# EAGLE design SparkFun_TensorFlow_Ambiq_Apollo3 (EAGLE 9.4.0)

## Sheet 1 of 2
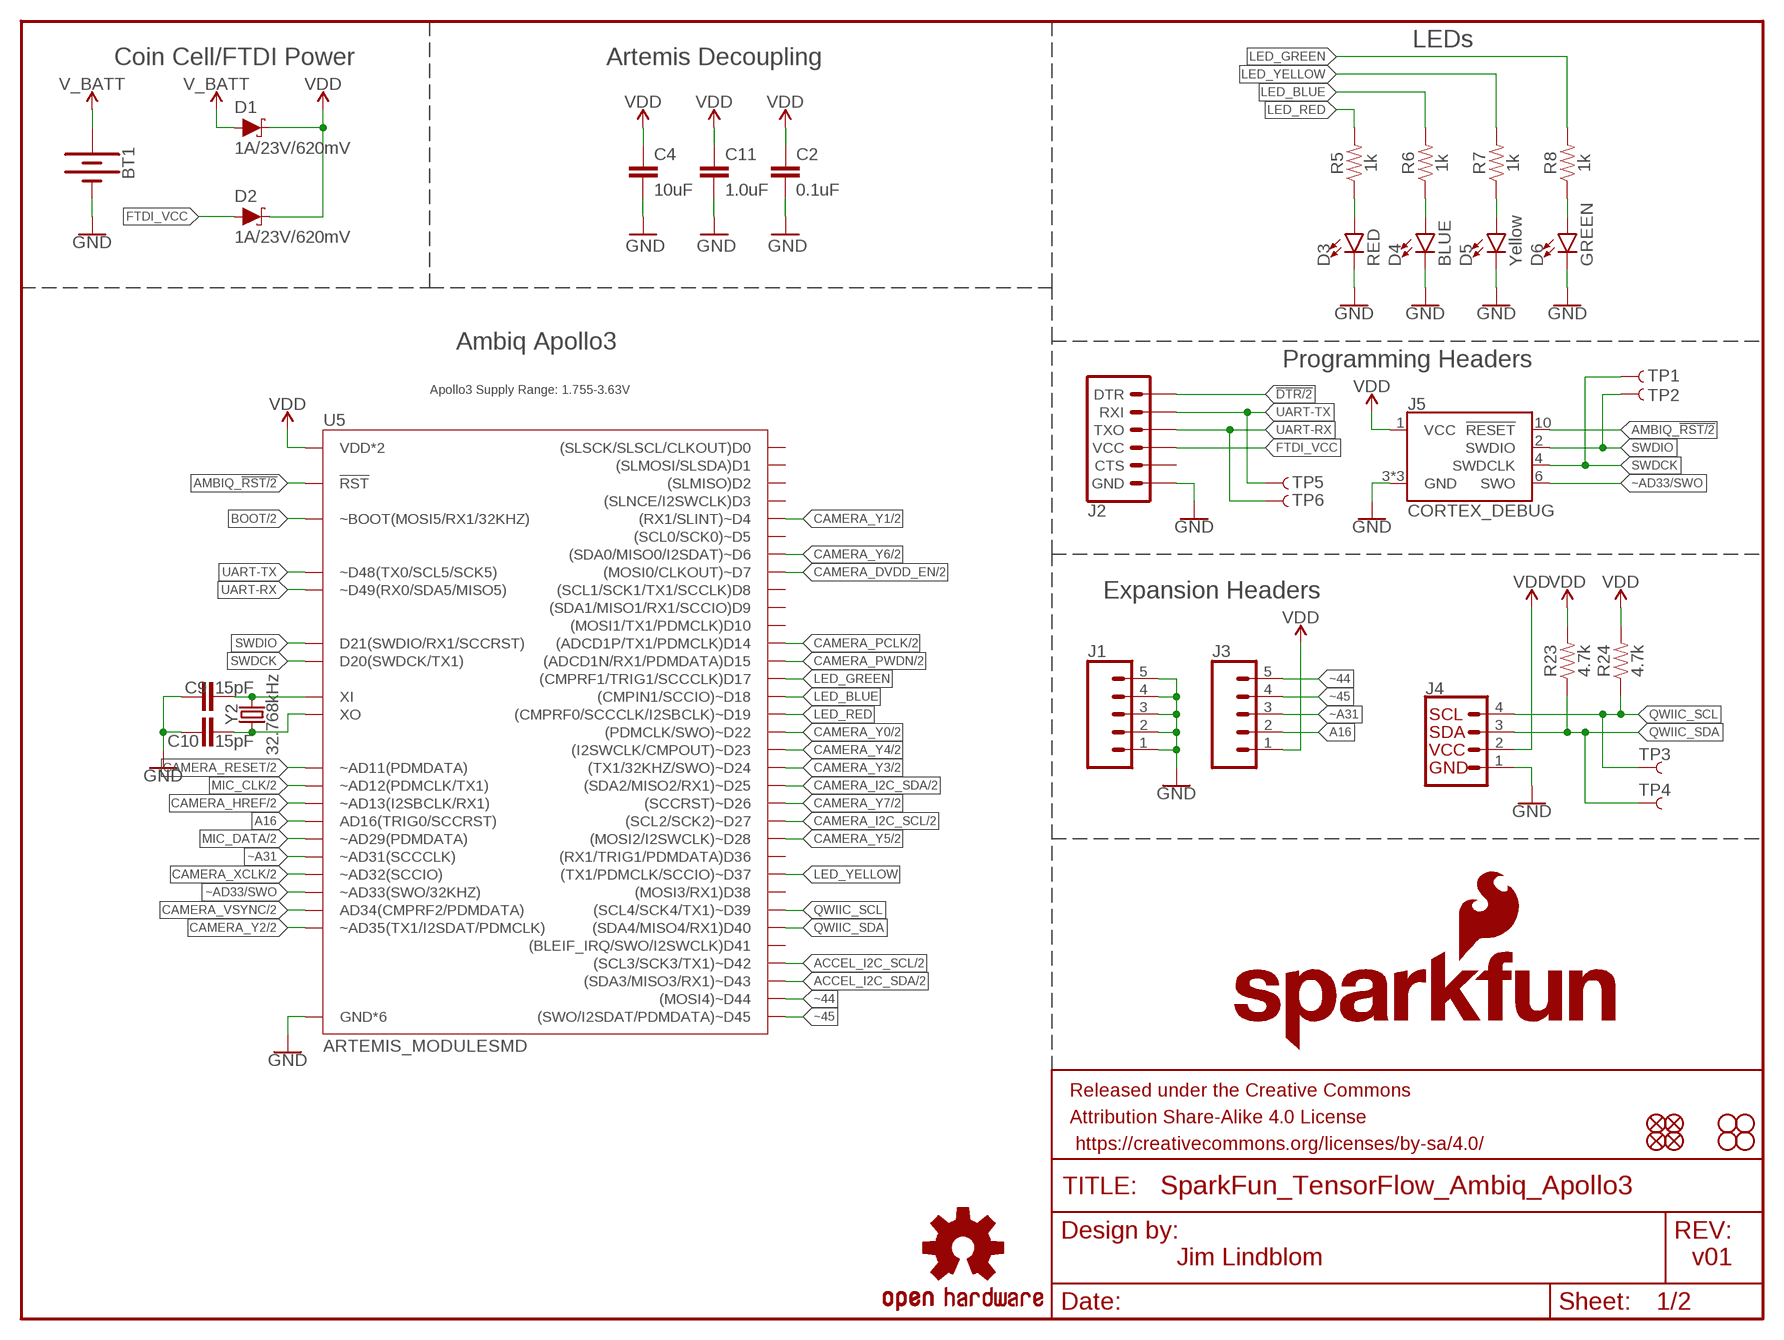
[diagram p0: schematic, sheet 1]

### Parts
BT1  BATTERY-20MM_SMD_4LEGS_OVERPASTE_INNER  [BATTCON_20MM_4LEGS_OVERPASTE_INNER]
C2  0.1uF  0.1UF-0402T-16V-10%  [0402-TIGHT]
C4  10uF  10UF-0603-6.3V-20%  [0603]
C9  15pF  15PF-0402-TIGHT-50V-5%  [0402-TIGHT]
C10  15pF  15PF-0402-TIGHT-50V-5%  [0402-TIGHT]
C11  1.0uF  1.0UF-0402T-16V-10%  [0402-TIGHT]
D1  1A/23V/620mV  DIODE-SCHOTTKY-BAT20J  [SOD-323]
D2  1A/23V/620mV  DIODE-SCHOTTKY-BAT20J  [SOD-323]
D3  RED  LED-RED0603  [LED-0603]
D4  BLUE  LED-BLUE0603  [LED-0603]
D5  Yellow  LED-YELLOW0603  [LED-0603]
D6  GREEN  LED-GREEN0603  [LED-0603]
FD1  FIDUCIAL1X2  [FIDUCIAL-1X2]
FD2  FIDUCIAL1X2  [FIDUCIAL-1X2]
FD3  FIDUCIAL1X2  [FIDUCIAL-1X2]
FD4  FIDUCIAL1X2  [FIDUCIAL-1X2]
FRAME1  FRAME-LETTER  [CREATIVE_COMMONS]
H1  STAND-OFF  [STAND-OFF]
H2  STAND-OFF  [STAND-OFF]
H3  STAND-OFF  [STAND-OFF]
H4  STAND-OFF  [STAND-OFF]
J1  CONN_05NO_SILK  [1X05_NO_SILK]
J2  6_PIN_SERIAL_TARGETSMD  [1X06-SMD_RA_MALE]
J3  CONN_05NO_SILK  [1X05_NO_SILK]
J4  QWIIC_CONNECTORJS-1MM  [JST04_1MM_RA]
J5  CORTEX_DEBUG  CORTEX_DEBUG_MINIMUM_PTH_NS  [2X5-PTH-1.27MM-NO_SILK]
LOGO1  SFE_LOGO_NAME_FLAME.1_INCH  [SFE_LOGO_NAME_FLAME_.1]
LOGO2  OSHW-LOGOS  [OSHW-LOGO-S]
R5  1k  1KOHM-0603-1/10W-1%  [0603]
R6  1k  1KOHM-0603-1/10W-1%  [0603]
R7  1k  1KOHM-0603-1/10W-1%  [0603]
R8  1k  1KOHM-0603-1/10W-1%  [0603]
R23  4.7k  4.7KOHM-0603-1/10W-1%  [0603]
R24  4.7k  4.7KOHM-0603-1/10W-1%  [0603]
TP1  TEST-POINT3X5  [PAD.03X.05]
TP2  TEST-POINT3X5  [PAD.03X.05]
TP3  TEST-POINT3X5  [PAD.03X.05]
TP4  TEST-POINT3X5  [PAD.03X.05]
TP5  TEST-POINT3X5  [PAD.03X.05]
TP6  TEST-POINT3X5  [PAD.03X.05]
U5  ARTEMIS_MODULESMD  [ARTEMIS_FP]
Y2  32.768kHz  CRYSTAL-32.768KHZSMD-3.2X1.5  [CRYSTAL-SMD-3.2X1.5MM]

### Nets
!DTR: J2.1(DTR) ; also sheet 2
A16: J3.2 U5.AD16(AD16(TRIG0/SCCRST))
ACCEL_I2C_SCL: U5.~D42((SCL3/SCK3/TX1)~D42) ; also sheet 2
ACCEL_I2C_SDA: U5.~D43((SDA3/MISO3/RX1)~D43) ; also sheet 2
AMBIQ_!RST: J5.10(!RESET) U5.~RST(!RST) ; also sheet 2
BOOT: U5.BOOT(~BOOT(MOSI5/RX1/32KHZ)) ; also sheet 2
CAMERA_DVDD_EN: U5.D7((MOSI0/CLKOUT)~D7) ; also sheet 2
CAMERA_HREF: U5.~AD13(~AD13(I2SBCLK/RX1)) ; also sheet 2
CAMERA_I2C_SCL: U5.~D27((SCL2/SCK2)~D27) ; also sheet 2
CAMERA_I2C_SDA: U5.~D25((SDA2/MISO2/RX1)~D25) ; also sheet 2
CAMERA_PCLK: U5.D14((ADCD1P/TX1/PDMCLK)D14) ; also sheet 2
CAMERA_PWDN: U5.D15((ADCD1N/RX1/PDMDATA)D15) ; also sheet 2
CAMERA_RESET: U5.~AD11(~AD11(PDMDATA)) ; also sheet 2
CAMERA_VSYNC: U5.AD34(AD34(CMPRF2/PDMDATA)) ; also sheet 2
CAMERA_XCLK: U5.~AD32(~AD32(SCCIO)) ; also sheet 2
CAMERA_Y0: U5.~D22((PDMCLK/SWO)~D22) ; also sheet 2
CAMERA_Y1: U5.~D4((RX1/SLINT)~D4) ; also sheet 2
CAMERA_Y2: U5.~AD35(~AD35(TX1/I2SDAT/PDMCLK)) ; also sheet 2
CAMERA_Y3: U5.~D24((TX1/32KHZ/SWO)~D24) ; also sheet 2
CAMERA_Y4: U5.~D23((I2SWCLK/CMPOUT)~D23) ; also sheet 2
CAMERA_Y5: U5.~D28((MOSI2/I2SWCLK)~D28) ; also sheet 2
CAMERA_Y6: U5.~D6((SDA0/MISO0/I2SDAT)~D6) ; also sheet 2
CAMERA_Y7: U5.~D26((SCCRST)~D26) ; also sheet 2
FTDI_VCC: D2.A J2.4(VCC)
GND: BT1.2(-) C2.1 C4.2 C9.1 C10.1 C11.2 D3.C D4.C D5.C D6.C J1.1 J1.2 J1.3 J1.4 J1.5 J2.6(GND) J4.1 J5.3(GND) J5.5(GND) J5.9(GND) U5.GND@1(GND*6) U5.GND@22(GND*6) U5.GND@38(GND*6) U5.GND@39(GND*6) U5.GND@47(GND*6) U5.GND@59(GND*6) ; also sheet 2
LED_BLUE: R6.2 U5.~D18((CMPIN1/SCCIO)~D18)
LED_GREEN: R8.2 U5.D17((CMPRF1/TRIG1/SCCCLK)D17)
LED_RED: R5.2 U5.~D19((CMPRF0/SCCCLK/I2SBCLK)~D19)
LED_YELLOW: R7.2 U5.~D37((TX1/PDMCLK/SCCIO)~D37)
MIC_CLK: U5.~AD12(~AD12(PDMCLK/TX1)) ; also sheet 2
MIC_DATA: U5.~AD29(~AD29(PDMDATA)) ; also sheet 2
N$2: C9.2 U5.XI Y2.P$2
N$5: D4.A R6.1
N$6: D3.A R5.1
N$7: D5.A R7.1
N$8: D6.A R8.1
QWIIC_SCL: J4.4 R24.1 TP3.P$1 U5.~D39((SCL4/SCK4/TX1)~D39)
QWIIC_SDA: J4.3 R23.1 TP4.P$1 U5.D40((SDA4/MISO4/RX1)D40)
SWDCK: J5.4(SWDCLK) TP1.P$1 U5.SWDCK(D20(SWDCK/TX1))
SWDIO: J5.2(SWDIO) TP2.P$1 U5.SWDIO(D21(SWDIO/RX1/SCCRST))
UART-RX: J2.3(TXO) TP6.P$1 U5.RXI-0(~D49(RX0/SDA5/MISO5))
UART-TX: J2.2(RXI) TP5.P$1 U5.TXO-0(~D48(TX0/SCL5/SCK5))
V_BATT: BT1.1(+) D1.A
VDD: C2.2 C4.1 C11.1 D1.C D2.C J3.1 J4.2 J5.1(VCC) R23.2 R24.2 U5.VDD@36(VDD*2) U5.VDD@37(VDD*2) ; also sheet 2
X0: C10.2 U5.XO Y2.P$1
~44: J3.5 U5.~D44((MOSI4)~D44)
~45: J3.4 U5.~D45((SWO/I2SDAT/PDMDATA)~D45)
~A31: J3.3 U5.~AD31(~AD31(SCCCLK))
~AD33/SWO: J5.6(SWO) U5.~AD33/SWO(~AD33(SWO/32KHZ))
Unconnected: J2.5(CTS) U5.D0((SLSCK/SLSCL/CLKOUT)D0) U5.D1((SLMOSI/SLSDA)D1) U5.D2((SLMISO)D2) U5.D3((SLNCE/I2SWCLK)D3) U5.D8((SCL1/SCK1/TX1/SCCLK)D8) U5.D9((SDA1/MISO1/RX1/SCCIO)D9) U5.D10((MOSI1/TX1/PDMCLK)D10) U5.D36((RX1/TRIG1/PDMDATA)D36) U5.D38((MOSI3/RX1)D38) U5.D41((BLEIF_IRQ/SWO/I2SWCLK)D41) U5.~D5((SCL0/SCK0)~D5)

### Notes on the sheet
- LEDs
- Coin Cell/FTDI Power | Artemis Decoupling
- Ambiq Apollo3
- Programming Headers
- Apollo3 Supply Range: 1.755-3.63V
- Expansion Headers
- Jim Lindblom | v01

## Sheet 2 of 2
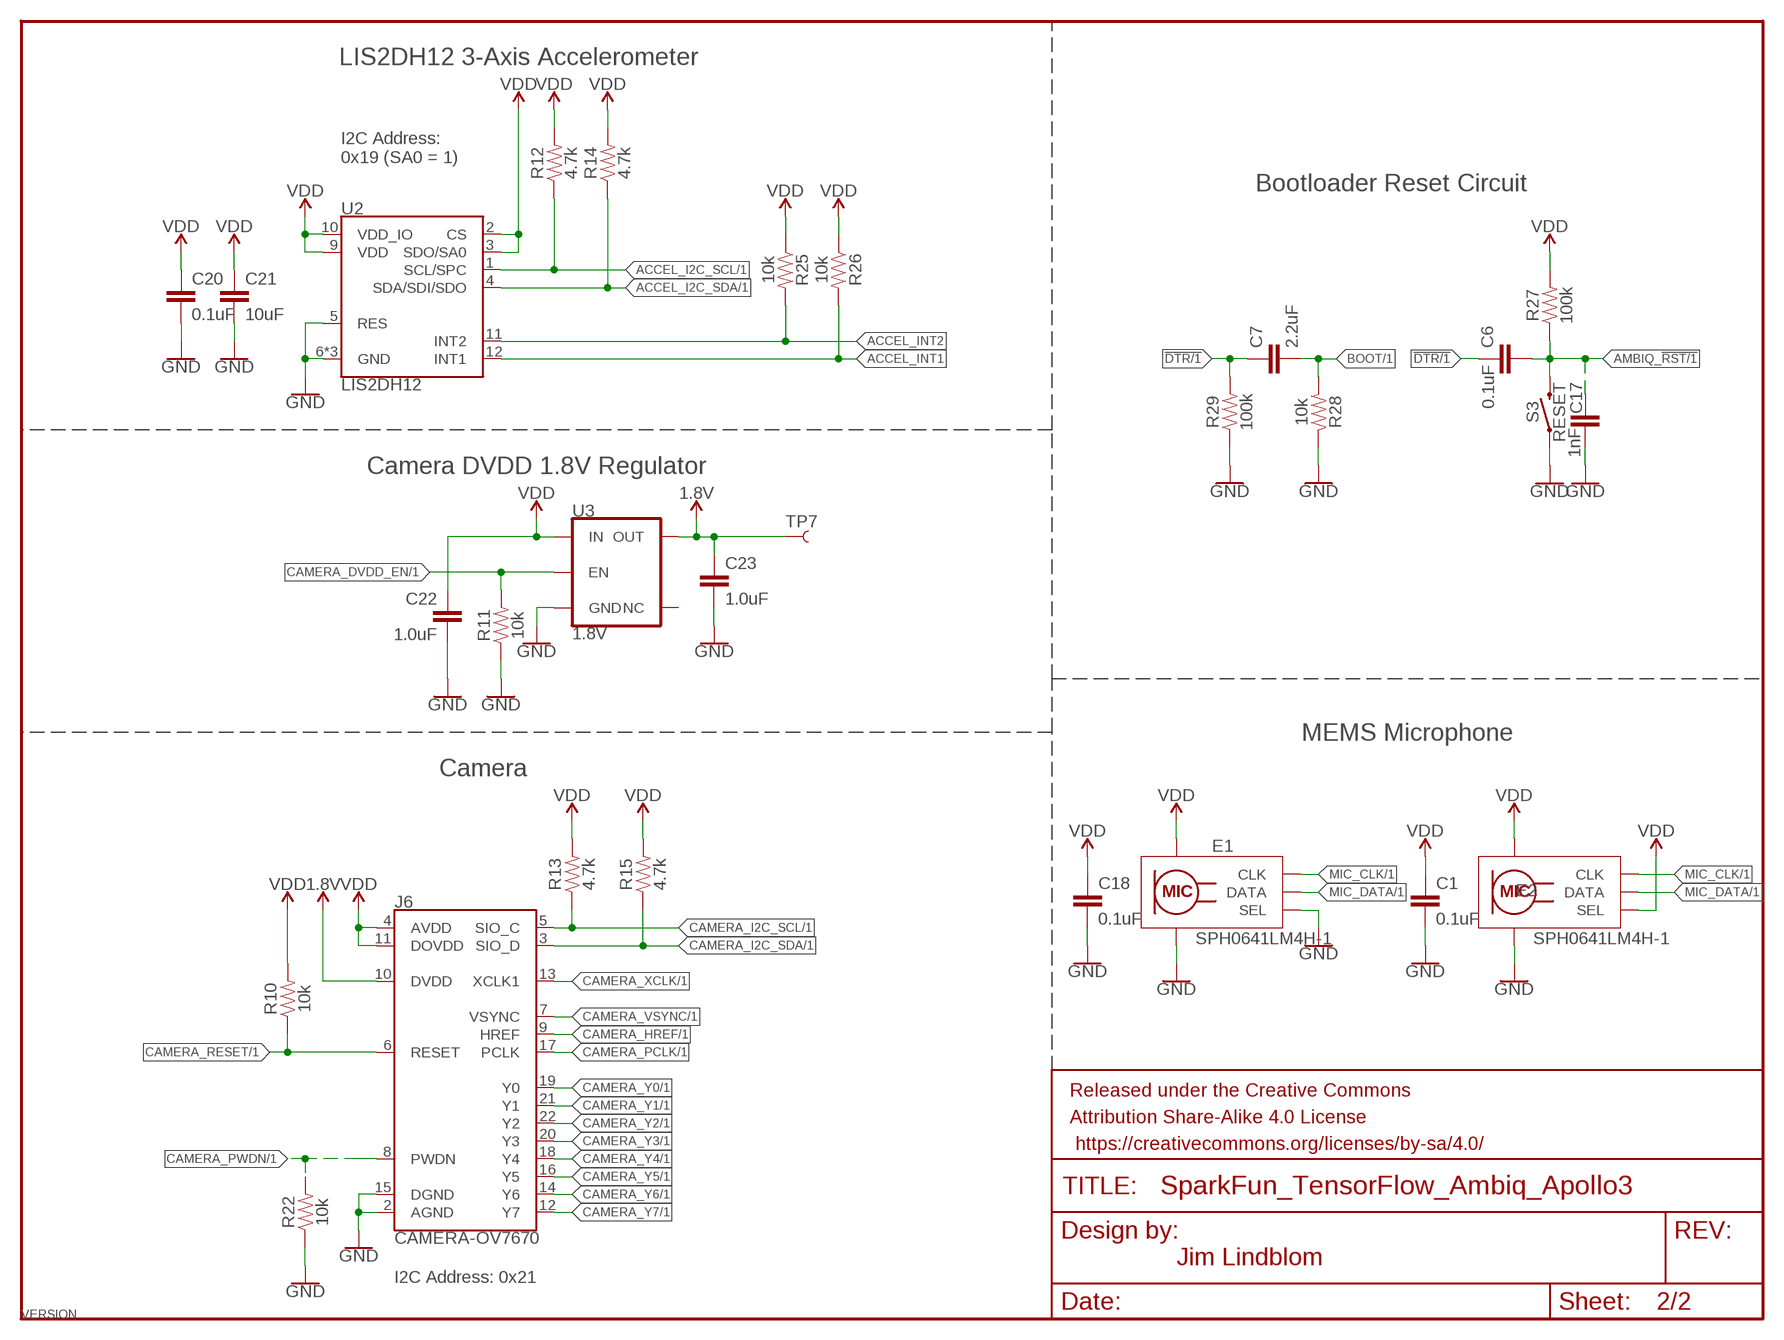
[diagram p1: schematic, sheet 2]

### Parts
C1  0.1uF  0.1UF-0402-TIGHT-16V-10%  [0402-TIGHT]
C6  0.1uF  0.1UF-0603-25V-5%  [0603]
C7  2.2uF  2.2UF-0603-10V-20%  [0603]
C17  1nF  1.0NF/1000PF-0603-50V-10%  [0603]
C18  0.1uF  0.1UF-0402-TIGHT-16V-10%  [0402-TIGHT]
C20  0.1uF  0.1UF-0402-TIGHT-16V-10%  [0402-TIGHT]
C21  10uF  10UF-0603-6.3V-20%  [0603]
C22  1.0uF  1.0UF-0402-TIGHT-16V-10%  [0402-TIGHT]
C23  1.0uF  1.0UF-0402-TIGHT-16V-10%  [0402-TIGHT]
E1  SPH0641LM4H-1  SPH0641LM4H-1_MICROPHONE  [SPH0641LM4H-1_MICROPHONE]
E2  SPH0641LM4H-1  SPH0641LM4H-1_MICROPHONE  [SPH0641LM4H-1_MICROPHONE]
FRAME2  FRAME-LETTERNO_PACKAGE  [DUMMY]
J6  CAMERA-OV7670  [FPC-24-AMPHENOL-SFV24R-1STE1HLF]
R10  10k  10KOHM-0402T-1/16W-1%  [0402-TIGHT]
R11  10k  10KOHM-0402T-1/16W-1%  [0402-TIGHT]
R12  4.7k  4.7KOHM-0603-1/10W-1%  [0603]
R13  4.7k  4.7KOHM-0603-1/10W-1%  [0603]
R14  4.7k  4.7KOHM-0603-1/10W-1%  [0603]
R15  4.7k  4.7KOHM-0603-1/10W-1%  [0603]
R22  10k  10KOHM-0402T-1/16W-1%  [0402-TIGHT]
R25  10k  10KOHM-0402T-1/16W-1%  [0402-TIGHT]
R26  10k  10KOHM-0402T-1/16W-1%  [0402-TIGHT]
R27  100k  100KOHM-0603-1/10W-1%  [0603]
R28  10k  10KOHM-0603-1/10W-1%  [0603]
R29  100k  100KOHM-0603-1/10W-1%  [0603]
S3  RESET  MOMENTARY-SWITCH-SPST-SMD-5.2MM-TALL  [TACTILE_SWITCH_SMD_5.2MM]
TP7  TEST-POINT3X5  [PAD.03X.05]
U2  LIS2DH12  [LGA-12-LISDH12]
U3  1.8V  V_REG_AP2127K-1.8V  [SOT23-5]

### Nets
1.8V: C23.1 J6.10(DVDD) TP7.P$1 U3.5(OUT)
!DTR: C6.1 C7.1 R29.2 ; also sheet 1
ACCEL_I2C_SCL: R12.1 U2.1(SCL/SPC) ; also sheet 1
ACCEL_I2C_SDA: R14.1 U2.4(SDA/SDI/SDO) ; also sheet 1
ACCEL_INT1: R26.2 U2.12(INT1)
ACCEL_INT2: R25.2 U2.11(INT2)
AMBIQ_!RST: C6.2 C17.1 R27.1 S3.3 ; also sheet 1
BOOT: C7.2 R28.2 ; also sheet 1
CAMERA_DVDD_EN: R11.2 U3.3(EN) ; also sheet 1
CAMERA_HREF: J6.9(HREF) ; also sheet 1
CAMERA_I2C_SCL: J6.5(SIO_C) R13.1 ; also sheet 1
CAMERA_I2C_SDA: J6.3(SIO_D) R15.1 ; also sheet 1
CAMERA_PCLK: J6.17(PCLK) ; also sheet 1
CAMERA_PWDN: J6.8(PWDN) R22.2 ; also sheet 1
CAMERA_RESET: J6.6(RESET) R10.1 ; also sheet 1
CAMERA_VSYNC: J6.7(VSYNC) ; also sheet 1
CAMERA_XCLK: J6.13(XCLK1) ; also sheet 1
CAMERA_Y0: J6.19(Y0) ; also sheet 1
CAMERA_Y1: J6.21(Y1) ; also sheet 1
CAMERA_Y2: J6.22(Y2) ; also sheet 1
CAMERA_Y3: J6.20(Y3) ; also sheet 1
CAMERA_Y4: J6.18(Y4) ; also sheet 1
CAMERA_Y5: J6.16(Y5) ; also sheet 1
CAMERA_Y6: J6.14(Y6) ; also sheet 1
CAMERA_Y7: J6.12(Y7) ; also sheet 1
GND: C1.2 C17.2 C18.2 C20.2 C21.2 C22.2 C23.2 E1.2(SEL) E1.3(GND) E1.6(GND) E1.7(GND) E1.8(GND) E2.3(GND) E2.6(GND) E2.7(GND) E2.8(GND) J6.2(AGND) J6.15(DGND) R11.1 R22.1 R28.1 R29.1 S3.1 U2.5(RES) U2.6(GND) U2.7(GND) U2.8(GND) U3.2(GND) ; also sheet 1
MIC_CLK: E1.4(CLK) E2.4(CLK) ; also sheet 1
MIC_DATA: E1.1(DATA) E2.1(DATA) ; also sheet 1
VDD: C1.1 C18.1 C20.1 C21.1 C22.1 E1.5(VDD) E2.2(SEL) E2.5(VDD) J6.4(AVDD) J6.11(DOVDD) R10.2 R12.2 R13.2 R14.2 R15.2 R25.1 R26.1 R27.2 U2.2(CS) U2.3(SDO/SA0) U2.9(VDD) U2.10(VDD_IO) U3.1(IN) ; also sheet 1
Unconnected: J6.MNT1@0(MNT1) J6.MNT1@1(MNT1) J6.MNT2@0(MNT2) J6.MNT2@1(MNT2) U3.4(NC)

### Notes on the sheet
- LIS2DH12 3-Axis Accelerometer
- I2C Address:
  0x19 (SA0 = 1)
- Bootloader Reset Circuit
- Camera DVDD 1.8V Regulator
- MEMS Microphone
- Camera
- Jim Lindblom
- I2C Address: 0x21

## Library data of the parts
BT1 = SparkFun-Batteries:BATTERY: Battery - Single Cell
C1 C18 C20 = ambiq:0.1UF: 0.1µF ceramic capacitors; PROD_ID: CAP-12416
C2 = SparkFun-Capacitors:0.1UF: 0.1µF ceramic capacitors; PROD_ID: CAP-12416
C4 C21 = SparkFun-Capacitors:10UF: 10.0µF ceramic capacitors; PROD_ID: CAP-11015
C6 = SparkFun-Capacitors:0.1UF: 0.1µF ceramic capacitors; PROD_ID: CAP-08604
C7 = SparkFun-Capacitors:2.2UF: 2.2µF ceramic capacitors; PROD_ID: CAP-07888
C9 C10 = ambiq:15PF: 15pF ceramic capacitors; PROD_ID: CAP-13063
C11 = SparkFun-Capacitors:1.0UF: 1µF ceramic capacitors; PROD_ID: CAP-12417
C17 = SparkFun-Capacitors:1.0NF/1000PF: 1nF/1,000pF ceramic capacitors; PROD_ID: CAP-07886
C22 C23 = ambiq:1.0UF: 1µF ceramic capacitors; PROD_ID: CAP-12417
D1 D2 = SparkFun-DiscreteSemi:DIODE-SCHOTTKY: Schottky diode; PROD_ID: DIO-11623
D3 = SparkFun-LED:LED-RED: Red SMD LED; PROD_ID: DIO-00819
D4 = SparkFun-LED:LED-BLUE: Blue SMD LED; PROD_ID: DIO-08575
D5 = SparkFun-LED:LED-YELLOW: Yellow SMD LED; PROD_ID: DIO-09003
D6 = SparkFun-LED:LED-GREEN: Green SMD LED; PROD_ID: DIO-00821
E1 E2 = SparkFun-Sensors:SPH0641LM4H-1_MICROPHONE: SPH0641LM4H-1 Microphone A miniature, high-performance, low power, bottom port silicon digital microphone with a single bit PDM output.; PROD_ID: IC-14361
FD1-FD4 = SparkFun-Aesthetics:FIDUCIAL: Fiducial Alignment Points
FRAME1 = SparkFun-Aesthetics:FRAME-LETTER: Schematic Frame - Letter
FRAME2 = SparkFun-Aesthetics:FRAME-LETTER: Schematic Frame - Letter; DESIGNER: Nobody; VERSION: x01
H1-H4 = SparkFun-Hardware:STAND-OFF: Stand Off
J1 J3 = SparkFun-Connectors:CONN_05: Multi connection point. Often used as Generic Header-pin footprint for 0.1 inch spaced/style header connections On any of the 0.1 inch spaced packages, you can populate with these: Break Away Headers - Straight (PRT-00116) Break Away Male Headers - Right Angle (PRT-00553) Female Headers (PRT-00115)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
J2 = SparkFun-Connectors:6_PIN_SERIAL_TARGET: 6-pin header connection for use with the "FTDI BASIC" pinout - TARGET SIDE. Also known as "Arduino Serial Program Header". It is used to mate with our FTDI Basic serial programmers using the Arduino IDE. Note, this device has "TARGET" in the name. It is intended to be used on a design that contains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; PROD_ID: CONN-08971
J4 = SparkFun-Connectors:QWIIC_CONNECTOR: SparkFun I2C Standard Qwiic Connector An SMD 1mm pitch JST connector makes it easy and quick (get it? Qwiic?) to connect I2C devices to each other. The Qwiic system enables fast and solderless connection between popular platforms and various sensors and actuators. We carry 200mm, 100mm, 50mm, and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; PROD_ID: CONN-13694
J5 = SparkFun-Connectors:CORTEX_DEBUG_MINIMUM: Cortex Debug Connector - 10 pin Supports JTAG debug, Serial Wire debug, and Serial Wire Viewer. PTH and SMD connector options available. General Connector Information Products: PTH Connector -via Digi-Key SparkFun PSoc SparkFun T
J6 = SparkFun-Connectors:CAMERA-OV7670; DIGIKEY: 609-4320-2-ND; PROD_ID: CONN-14233
LOGO1 = SparkFun-Aesthetics:SFE_LOGO_NAME_FLAME: SparkFun Font Logo w/ Flame
LOGO2 = SparkFun-Aesthetics:OSHW-LOGO: Open-Source Hardware (OSHW) Logo
R5-R8 = SparkFun-Resistors:1KOHM: 1kΩ resistor; PROD_ID: RES-07856
R10 R11 R22 R25 R26 = SparkFun-Resistors:10KOHM: 10kΩ resistor; PROD_ID: RES-14241
R12-R15 R23 R24 = SparkFun-Resistors:4.7KOHM: 4.7kΩ resistor; PROD_ID: RES-07857
R27 R29 = SparkFun-Resistors:100KOHM: 100kΩ resistor; PROD_ID: RES-07828
R28 = SparkFun-Resistors:10KOHM: 10kΩ resistor; PROD_ID: RES-00824
S3 = SparkFun-Switches:MOMENTARY-SWITCH-SPST: Momentary Switch (Pushbutton) - SPST; PROD_ID: SWCH-14139
TP1-TP7 = SparkFun-Connectors:TEST-POINT: SparkFun Test Points
U2 = SparkFun-Sensors:LIS2DH12; DIGIKEY: 497-14851-2-ND; PROD_ID: IC-14229
U3 = SparkFun-IC-Power:V_REG_AP2127: AP2127 - 300mA CMOS LDO Regulator w/ Enable The AP2127 is CMOS process low dropout linear regulator with enable function, the regulator delivers a guaranteed 300mA (min.) continuous load current. Features Output Voltage Accuracy: ±1.5% Output Current: 300mA (Min.) Foldback Short Current Protection: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; PROD_ID: VREG-14239
U5 = Testing:ARTEMIS_MODULE
Y2 = SparkFun-Clocks:CRYSTAL-32.768KHZ: 32.768kHz Crystal; PROD_ID: XTAL-13062

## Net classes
0 default: width 0 mm, drill 0 mm
2 usb: width 0.254 mm, drill 0.305 mm, clearance 0.254 mm

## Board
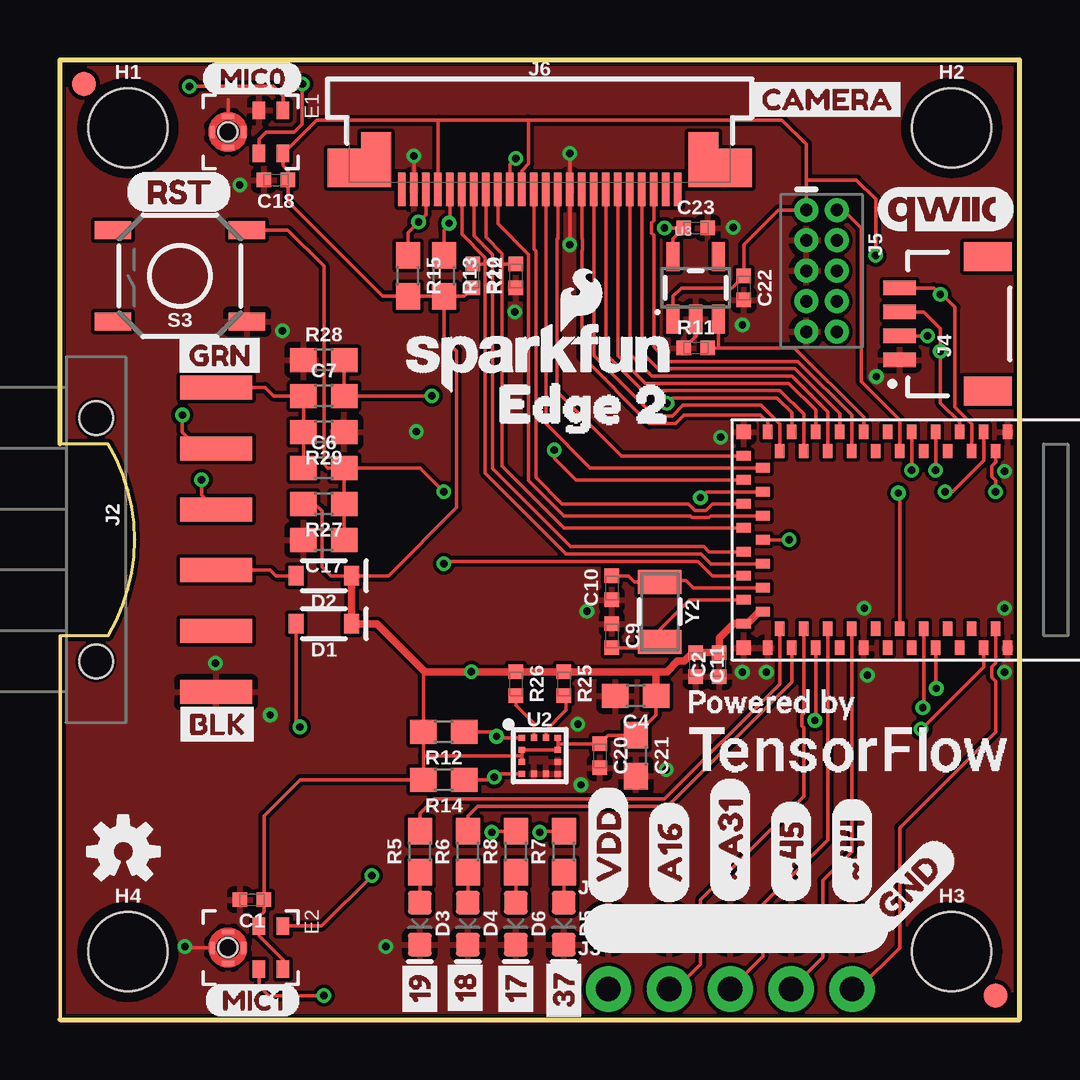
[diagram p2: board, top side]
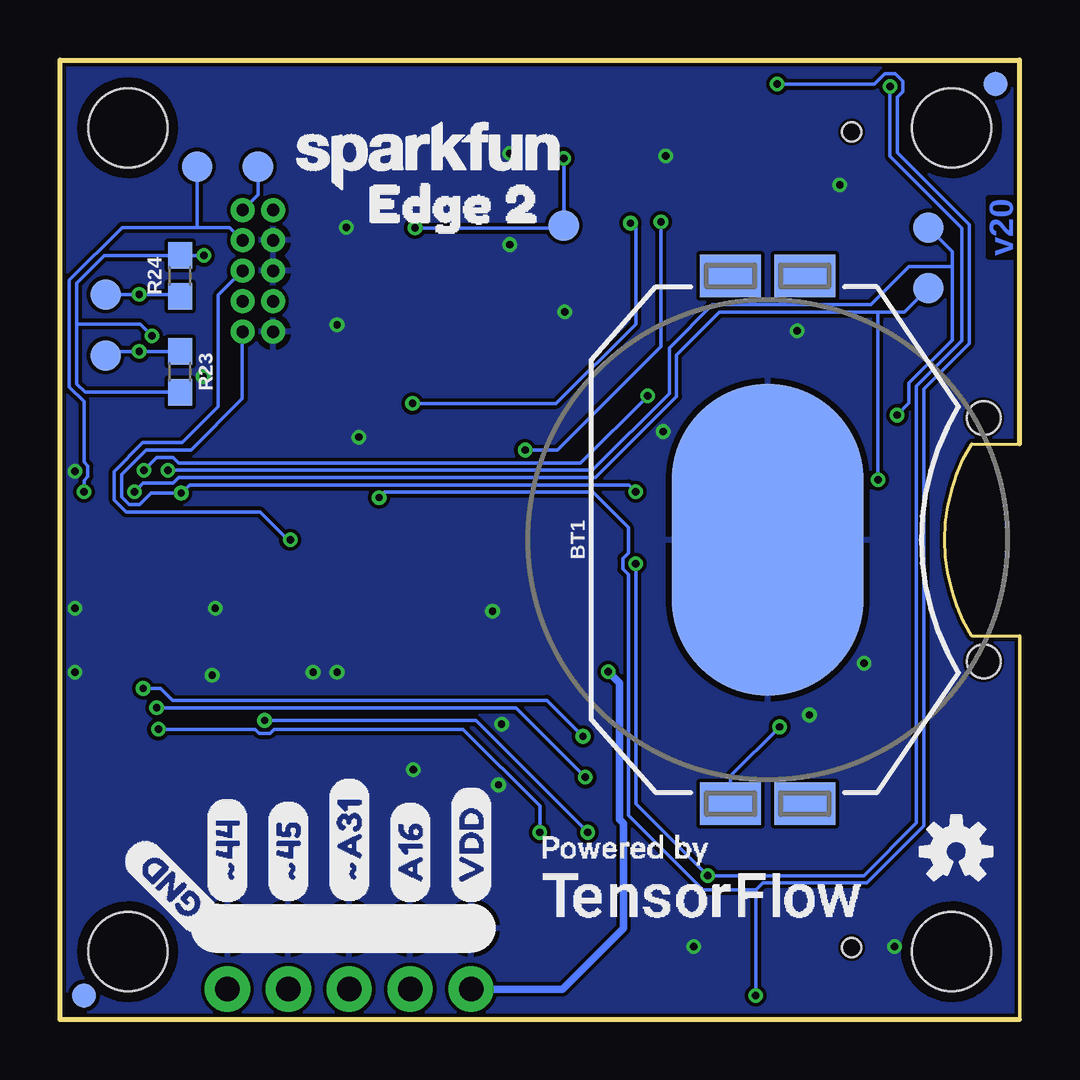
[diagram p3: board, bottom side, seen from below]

Size 40 x 40 mm. Coordinates in mm from the lower left corner, seen from the top.
Outline: 0,0 40,0 40,40 0,40 0,24 2,24 arc-62 2,16 0,16 0,0
Copper layers (1*16): Top 0.035mm / dielectric 1.5mm / Bottom 0.035mm
Design rules "SparkFun-2-layer-PCBWay-LIMIT *": minimum track width 6mil, minimum drill 0.3mm, track to track 6mil, track to pad 6mil, pad to pad 6mil, via to via 6mil, smd to smd 6mil, copper to edge 6mil, drill to drill 6mil, minimum pad ring 6mil, minimum via ring 6mil, stop-mask expansion 4mil, vias tented up to drill 25mil, thermal gap 10mil

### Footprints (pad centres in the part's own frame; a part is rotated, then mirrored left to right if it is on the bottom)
BATTCON_20MM_4LEGS_OVERPASTE_INNER = smd 1.778 x 2.54: 1 -11,1.55; 3 11,1.55; P$1 -11,-1.55; P$2 11,-1.55 | smd 13 x 8: 2 0,0
0402-TIGHT = smd 0.6 x 0.6: 1 -0.5,0; 2 0.5,0
0603 = smd 1.1 x 1: 1 -0.85,0; 2 0.85,0
SOD-323 = smd 0.63 x 0.83: A 1.15,0; C -1.15,0
LED-0603 = smd 1 x 1: A -0.877,0; C 0.877,0
SPH0641LM4H-1_MICROPHONE = smd 0.725 x 0.522: 1 -0.9,1.3; 2 -0.9,0.3; 4 0.9,0.3; 5 0.9,1.3 | smd 0.5 x 0.2: 3 0,-1.65; 8 0,-0.35 | smd 0.2 x 0.5: 6 -0.65,-1; 7 0.65,-1 | hole 0.8: 0,-1
FIDUCIAL-1X2 = smd 1 x 1: 1 0,0
STAND-OFF = hole 3.302: 0,0
1X05_NO_SILK = drill 1.016 pad 1.88: 1 0,0; 2 2.54,0; 3 5.08,0; 4 7.62,0; 5 10.16,0
1X06-SMD_RA_MALE = smd 1 x 3: 1 -6.35,5; 2 -3.81,5; 3 -1.27,5; 4 1.27,5; 5 3.81,5; 6 6.35,5 | hole 1.4: -5.08,0; 5.08,0
JST04_1MM_RA = smd 0.6 x 1.35: 1 -1.5,0; 2 -0.5,0; 3 0.5,0; 4 1.5,0 | smd 1.2 x 2: NC1 2.8,-3.675; NC2 -2.8,-3.675
2X5-PTH-1.27MM-NO_SILK = drill 0.508 pad 1: 1 -2.54,-0.635; 2 -2.54,0.635; 3 -1.27,-0.635; 4 -1.27,0.635; 5 0,-0.635; 6 0,0.635; 7 1.27,-0.635; 8 1.27,0.635; 9 2.54,-0.635; 10 2.54,0.635
FPC-24-AMPHENOL-SFV24R-1STE1HLF = smd 0.3 x 1.4: 1 5.75,2.4; 2 5.25,2.4; 3 4.75,2.4; 4 4.25,2.4; 5 3.75,2.4; 6 3.25,2.4; 7 2.75,2.4; 8 2.25,2.4; 9 1.75,2.4; 10 1.25,2.4; 11 0.75,2.4; 12 0.25,2.4; 13 -0.25,2.4; 14 -0.75,2.4; 15 -1.25,2.4; 16 -1.75,2.4; 17 -2.25,2.4; 18 -2.75,2.4; 19 -3.25,2.4; 20 -3.75,2.4; 21 -4.25,2.4; 22 -4.75,2.4; 23 -5.25,2.4; 24 -5.75,2.4 | smd 1.4 x 1.6: MNT1@0 -8.15,1.5; MNT2@1 8.15,1.5 | smd 1.25 x 2.3: MNT1@1 -6.825,1.15; MNT2@0 6.825,1.15
TACTILE_SWITCH_SMD_5.2MM = smd 1.524 x 0.762: 1 -2.794,1.905; 2 2.794,1.905; 3 -2.794,-1.905; 4 2.794,-1.905
PAD.03X.05 = smd 1.27 x 1.27: P$1 0,0
LGA-12-LISDH12 = smd 0.275 x 0.25: 1 -0.75,0.75; 2 -0.75,0.25; 3 -0.75,-0.25; 4 -0.75,-0.75; 7 0.75,-0.75; 8 0.75,-0.25; 9 0.75,0.25; 10 0.75,0.75 | smd 0.25 x 0.275: 5 -0.25,-0.75; 6 0.25,-0.75; 11 0.25,0.75; 12 -0.25,0.75
SOT23-5 = smd 0.55 x 1.2: 1 -0.95,-1.3; 2 0,-1.3; 3 0.95,-1.3; 4 0.95,1.3; 5 -0.95,1.3
ARTEMIS_FP = smd 0.4 x 0.6: AD16 -4,-3.7; BOOT 1.5,4.5; D0 0.5,-4.5; D1 -0.5,-4.5; D2 -1,-3.7; D3 2,-3.7; D7 -1.5,4.5; D8 -0.5,4.5; D9 2,3.7; D10 1,3.7; D14 -5,3.7; D17 -3.5,-4.5; D36 2.5,-4.5; D38 3,-3.7; D40 2.5,4.5; D41 -2.5,-4.5; GND@1 4.5,4.5; GND@39 -5.5,-4.5; GND@47 -1.5,-4.5; GND@59 4.5,-4.5; RXI-0 3.5,4.5; SWDCK 4,3.7; SWDIO 0,3.7; TXO-0 0.5,4.5; ~AD31 -3,-3.7; ~AD35 -2,3.7; ~D4 -2.5,4.5; ~D5 -1,3.7; ~D18 -4.5,-4.5; ~D19 -5,-3.7; ~D22 -3.5,4.5; ~D23 -4,3.7; ~D24 -3,3.7; ~D27 -4.5,4.5; ~D28 -5.5,4.5; ~D37 3.5,-4.5; ~D39 3,3.7; ~D42 1.5,-4.5; ~D43 1,-3.7; ~D44 4,-3.7; ~D45 -2,-3.7; ~RST 0,-3.7 | smd 0.6 x 0.4: AD34 -6.5,-0.5; D15 -6.5,0.5; VDD@36 -5.7,-3; VDD@37 -6.5,-3.5; XI -6.5,-2.5; XO -5.7,-2; ~AD11 -5.7,-1; ~AD12 -5.7,2; ~AD13 -5.7,1; ~AD29 -6.5,-1.5; ~AD32 -5.7,3; ~AD33/SWO -5.7,0; ~D6 -6.5,3.5; ~D25 -6.5,2.5; ~D26 -6.5,1.5 | smd 0.6 x 0.6: GND@22 -6.5,4.5; GND@38 -6.5,-4.5
CRYSTAL-SMD-3.2X1.5MM = smd 1 x 1.8: P$1 -1.25,0; P$2 1.25,0

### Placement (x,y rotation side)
BT1  10.5,20 90 bottom
C1  8,5 180 top
C2  27.48,14.8 90 top
C4  24,13.5 180 top
C6  11,23 0 top
C7  11,26 0 top
C9  23,16 270 top
C10  23,18 90 top
C11  26.51,14.8 270 top
C17  11,20 180 top
C18  9,35 180 top
C20  22.5,11 270 top
C21  24,11 270 top
C22  28.5,30.5 270 top
C23  26.5,33 0 top
D1  11,16.5 180 top
D2  11,18.5 180 top
D3  15,4 270 top
D4  17,4 270 top
D5  21,4 270 top
D6  19,4 270 top
E1  8,37 270 top
E2  8,3 270 top
FD1  1,39 0 top
FD2  39,1 0 top
FD3  39,1 0 bottom
FD4  1,39 0 bottom
FRAME1  not placed on the board
FRAME2  not placed on the board
H1  2.83,37.17 0 top
H2  37.17,37.17 0 top
H3  37.17,2.83 0 top
H4  2.83,2.83 0 top
J1  22.86,3.81 0 top
J2  1.5,20 270 top
J3  22.86,1.27 0 top
J4  35,29 90 top
J5  31.75,31.21 270 top
J6  20,37 180 top
LOGO1  20,27.6 0 top
LOGO2  2.64,7 0 top
R5  15,7 90 top
R6  17,7 90 top
R7  21,7 90 top
R8  19,7 90 top
R10  17.2,31 270 top
R11  26.5,28 0 top
R12  16,12 180 top
R13  16,31 270 top
R14  16,10 180 top
R15  14.5,31 270 top
R22  19,31 90 top
R23  35,27 270 bottom
R24  35,31 90 bottom
R25  21,14 270 top
R26  19,14 270 top
R27  11,21.5 180 top
R28  11,27.5 0 top
R29  11,24.5 180 top
S3  5,31 180 top
TP1  34.29,35.56 0 bottom
TP2  31.75,35.56 0 bottom
TP3  38.1,30.23 0 bottom
TP4  38.1,27.69 0 bottom
TP5  3.81,33.02 0 bottom
TP6  3.81,30.48 0 bottom
TP7  19,33.1 0 bottom
U2  20,11 0 top
U3  26.5,30.5 0 top
U5  35,20 0 top
U$1  [MIC00]  5.92,39.24 0 top
U$2  [BLK2]  4.57,12.32 0 top
U$3  [GND0]  33.66,3.81 45 top
U$4  [VDD1]  22.86,4.83 90 top
U$5  [#453]  30.48,4.83 90 top
U$6  [#A312]  27.94,4.83 90 top
U$7  [A161]  25.4,4.83 90 top
U$8  [MIC10]  6,0.8 0 top
U$9  [VDD1]  22.86,4.83 90 bottom
U$10  [A161]  25.4,4.83 90 bottom
U$11  [#A312]  27.94,4.83 90 bottom
U$12  [#453]  30.48,4.83 90 bottom
U$13  [#444]  33.02,4.83 90 bottom
U$14  [GND0]  33.66,3.81 135 bottom
U$15  [EDGE_20]  16.89,25.65 0 top
U$16  [372]  21,-0.3 90 top
U$19  [QWIIC_COPYRIGHT_SMALL]  36.9,33.8 0 top
U$20  [CAMERA3]  28.45,38.35 0 top
U$21  [POWEREDBY_TF#JPG]  32.77,12.3 0 top
U$23  [171]  19,-0.1 90 top
U$25  [POWEREDBY_TF#JPG]  13.34,6.22 0 bottom
U$26  [182]  16.9,-0.1 90 top
U$27  [RST15]  2.7,34.5 0 top
U$28  [GRN1]  4.57,27.69 0 top
U$29  [SFE_LOGO_NAME_.1]  24.64,36 0 bottom
U$30  [OSHW-LOGO-S]  2.64,7 0 bottom
U$31  [193]  15,-0.1 90 top
U$32  [EDGE_20]  28.54,34 0 bottom
U$36  [#444]  33.02,4.83 90 top
Y2  25,17 270 top

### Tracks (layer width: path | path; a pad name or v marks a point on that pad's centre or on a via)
1.8V  (via drill 0.3)
  Top 0.152: U3.5 25.55,32.55 C23.1 v25.2,33 | J6.10 18.75,35.65 v19,35.9
  Bottom 0.152: v25.2,33 19.1,33 TP7.P$1 v19,35.9
!DTR
  Top 0.152: J2.1 8.55,26.35 8.9,26 C7.1 R29.2 C6.1
A16
  Top 0.152: J3.2 25.67,1.27 26.7,2.3 26.7,5 31,9.3 31,12.18 30.93,12.25 30.93,12.69 31,12.75 U5.AD16
ACCEL_I2C_SCL  (via drill 0.3)
  Top 0.152: U2.1 18.25,11.75 v18.2,11.8 18,12 R12.1 | U5.~D42 36.5,13.83 v36.53,13.8
  Bottom 0.152: v36.53,13.8 35.8,13.8 35.3,13.3 19.7,13.3 v18.2,11.8
ACCEL_I2C_SDA  (via drill 0.3)
  Top 0.152: U2.4 18.25,10.25 v18.1,10.1 18,10 R14.1 | U5.~D43 36,13.03 v35.97,13
  Bottom 0.152: v35.97,13 21,13 v18.1,10.1
ACCEL_INT1
  Top 0.152: U2.12 19.75,12.35 19,13.1 R26.2
ACCEL_INT2
  Top 0.152: U2.11 20.25,12.05 21.1,12.9 21.1,13.4 R25.2
AMBIQ_!RST  (via drill 0.3)
  Top 0.152: C17.1 R27.1 11.85,22.95 11.8,23 | v16,22 15,23 C6.2 11.8,23 | v34.95,21.95 35,21.89 U5.~RST | S3.3 9.49,32.91 11,31.4 11,23.15 11.15,23 11.8,23
  Bottom 0.152: J5.10 32.4,28.66 32.4,25.88 34.54,23.74 36.42,23.74 37.43,22.72 37.43,21.78 37.12,21.47 36.68,21.47 36.2,21.95 v34.95,21.95 34.6,22.29 16.29,22.29 v16,22
BOOT  (via drill 0.3)
  Top 0.152: R28.2 C7.2 v15.5,26 | U5.BOOT v36.5,22.9
  Bottom 0.152: v36.5,22.9 35.97,23.43 35.28,23.43 35.05,23.2 18.3,23.2 v15.5,26
CAMERA_DVDD_EN
  Top 0.152: U5.D7 33.5,25.12 30.62,28 27.4,28 | 27.4,28 R11.2 | U3.3 27.45,28.05 27.4,28
CAMERA_HREF
  Top 0.152: J6.9 18.25,33.17 19.53,31.89 19.53,22.47 21,21 26.27,21 26.35,20.92 27.05,20.92 27.13,21 U5.~AD13
CAMERA_I2C_SCL  (via drill 0.3)
  Top 0.152: U5.~D27 30.5,25.3 29.89,25.91 25.53,25.91 v25.3,25.68 | J6.5 16.25,33.17 | R13.1 16,32.9 16.25,33.15 16.25,33.17 | v16.22,33.2 16.25,33.17
  Bottom 0.152: v25.3,25.68 19.32,25.68 16,29 16,32.98 v16.22,33.2
CAMERA_I2C_SDA  (via drill 0.3)
  Top 0.152: U5.~D25 21.5,22.5 20.61,23.39 v20.61,23.74 | J6.3 15.25,33.55 v14.95,33.25 14.5,32.8 R15.1
  Bottom 0.152: v20.61,23.74 19.26,23.74 14.95,28.05 v14.95,33.25
CAMERA_PCLK
  Top 0.152: J6.17 22.25,27.68 24.78,25.15 25.52,25.15 25.98,25.61 29.23,25.61 30,24.83 U5.D14
CAMERA_PWDN
  Top 0.152: U5.D15 21,20.5 18.43,23.07 18.43,29.73 18.43,31.5 | J6.8 17.75,32.6 18.43,31.92 18.43,31.5 | R22.2 18.43,31.5
CAMERA_RESET
  Top 0.152: U5.~AD11 27.13,19 26.73,19.41 21.09,19.41 17.72,22.78 17.72,23.1 17.73,23.1 17.73,31.5 | J6.6 16.75,32.74 17.73,31.76 17.73,31.5 | R10.1 17.73,31.5
CAMERA_VSYNC
  Top 0.152: U5.AD34 27.06,19.5 26.85,19.71 21.29,19.71 18.03,22.97 18.03,31.89 17.25,32.67 J6.7
CAMERA_XCLK
  Top 0.152: U5.~AD32 22.1,23 20.25,24.85 J6.13
CAMERA_Y0
  Top 0.152: U5.~D22 31.5,25.4 30.38,26.52 24.41,26.52 23.25,27.68 J6.19
CAMERA_Y1
  Top 0.152: U5.~D4 32.5,25.26 30.63,27.13 24.92,27.13 24.25,27.8 J6.21
CAMERA_Y2
  Top 0.152: U5.~AD35 33,25.19 30.76,27.43 25.37,27.43 24.85,27.95 24.75,28.05 24.75,32.7 24.67,32.78 24.67,33.22 24.75,33.3 J6.22
CAMERA_Y3
  Top 0.152: U5.~D24 32,25.33 30.51,26.82 24.68,26.82 23.75,27.75 J6.20
CAMERA_Y4
  Top 0.152: U5.~D23 31,25.23 30.02,26.21 24.29,26.21 22.75,27.75 J6.18
CAMERA_Y5
  Top 0.152: U5.~D28 29.5,24.9 29.2,25.2 26,25.2 25.65,24.84 24.56,24.84 21.75,27.65 21.75,32.05 21.78,32.08 21.78,32.52 21.75,32.55 J6.16
CAMERA_Y6
  Top 0.152: U5.~D6 23.4,23.5 20.72,26.18 20.72,32.52 20.75,32.55 J6.14
CAMERA_Y7
  Top 0.152: J6.12 19.75,32.1 19.83,32.02 19.83,22.6 20.93,21.5 26.2,21.5 26.48,21.22 26.92,21.22 27.2,21.5 U5.~D26
FTDI_VCC
  Top 0.152: J2.4 8.77,18.73 9,18.5 D2.A
GND  (via drill 0.3)
  Top 0.152: 34.3,26.8 v34.03,26.8 | J6.2 v14.75,36 | v21.25,36.1 J6.15 v21.25,32.3 | 6.37,3.02 E2.3 5.25,3 v5.21,3.05 | 6.37,3.02 6.37,3.26 6.74,3.63 6.98,3.63 E2.6 7.02,3.63 7.26,3.63 7.63,3.26 7.63,3.02 E2.8 7.63,2.98 7.63,2.74 7.26,2.37 7.02,2.37 E2.7 6.98,2.37 6.74,2.37 6.37,2.74 6.37,3.02 | E1.6 6.98,37.63 6.74,37.63 6.37,37.26 6.37,37.02 E1.3 6.37,36.98 6.37,36.74 6.74,36.37 6.98,36.37 E1.7 7.02,36.37 7.26,36.37 7.63,36.74 7.63,36.98 E1.8 7.63,37.02 7.63,37.26 7.26,37.63 7.02,37.63 E1.6 | E1.6 7,38.35 | U3.2 26.5,28.5 R11.1
  other vias: 13.59,3.05 6.48,14.86 8.76,12.7 21.97,17.02 28.45,14.48 33.66,14.35 33.53,17.14 39.37,22.86 39.37,17.14 39.37,14.48 28.45,28.96 28.07,33.02 7.49,34.8 9.27,28.7 14.86,24.51 21.72,9.78 25.27,10.41 21.59,12.32 18.96,29.51 29.45,14.48 27.55,24.28
  pour Bottom (isolate 0.152): 0,40 0,0 40,0 40,40
  pour Top (isolate 0.152): 0,40 40,40 40,0 0,0
LED_BLUE
  Top 0.152: U5.~D18 30.5,14.07 25.33,8.89 17.4,8.89 17,8.49 R6.2
LED_GREEN  (via drill 0.3)
  Top 0.152: U5.D17 31.5,12.5 v31.47,12.47 | v18,7.8 18.05,7.85 R8.2
  Bottom 0.152: v31.47,12.47 22.67,12.47 v18,7.8
LED_RED
  Top 0.152: U5.~D19 30,14 25.2,9.2 15.6,9.2 15,8.6 R5.2
LED_YELLOW  (via drill 0.3)
  Top 0.152: U5.~D37 38.5,14.7 v35.9,12.1 | v20,7.8 20.05,7.85 R7.2
  Bottom 0.152: v35.9,12.1 31.85,12.1 31.69,11.93 31.25,11.93 31.08,12.1 23.2,12.1 20,8.9 v20,7.8
MIC_CLK  (via drill 0.3)
  Top 0.152: E2.4 8.3,1.4 8.7,1 v11,1 | v26.7,21.76 26.94,22 U5.~AD12 | E1.4 8.3,36.7 8.6,37 9.77,37 10.1,37.33 v10.1,39
  Bottom 0.152: v26.7,21.76 26.47,21.99 17.79,21.99 16.3,20.5 16.3,19.45 16.53,19.22 16.53,18.78 16.3,18.55 16.3,8.51 13.2,5.4 11,5.4 | v10.1,39 6.05,39 5.62,39.43 5.18,39.43 4.87,39.12 4.87,38.68 5.09,38.45 5.09,36.13 2.1,33.13 2.1,28.17 4,26.27 4,8.07 6.37,5.7 10.71,5.7 11,5.4 | v11,1 11,5.4
MIC_DATA  (via drill 0.3)
  Top 0.152: U5.~AD29 27.2,18.5 26.6,19.1 16.1,19.1 v16,19 | E2.1 10.9,3.9 v13,6 | E1.1 9.3,38.5 8.9,38.9 v5.4,38.9
  Bottom 0.152: v16,19 16,9 v13,6 6.5,6 4.3,8.2 4.3,26.4 2.4,28.3 2.4,33 5.4,36 v5.4,38.9
N$2
  Top 0.152: U5.XI 26.23,17.5 25,16.27 Y2.P$2 24.75,15.5 C9.2
N$5
  Top 0.152: R6.1 D4.A
N$6
  Top 0.152: R5.1 D3.A
N$7
  Top 0.152: R7.1 D5.A
N$8
  Top 0.152: R8.1 D6.A
QWIIC_SCL  (via drill 0.3)
  Top 0.152: J4.4 36.43,30.5 v36.7,30.23 36.77,30.23 37.3,29.7 37.3,25.53 38,24.83 U5.~D39
  Bottom 0.152: R24.1 35.08,30.23 v36.7,30.23 TP3.P$1
QWIIC_SDA  (via drill 0.3)
  Top 0.152: J4.3 36,29.5 36.7,28.8 v36.7,27.85 36.7,25.7 37.5,24.9 U5.D40
  Bottom 0.152: R23.1 v36.7,27.85 37.94,27.85 TP4.P$1
SWDCK  (via drill 0.3)
  Top 0.152: U5.SWDCK 39,23.24 38.84,23.08 38.84,22.64 39,22.48 v39,22
  Bottom 0.152: v39,22 39,22.48 38.84,22.64 38.84,23.08 39,23.24 39,25.77 39.6,26.37 39.6,30.83 37.41,33.02 34.29,33.02 | J5.4 32.92,33.02 34.29,33.02 | TP1.P$1 34.29,33.02
SWDIO
  Top 0.152: U5.SWDIO 35,25 33.4,26.6 33.4,33 32.65,33.75 J5.2
  Bottom 0.152: J5.2 31.75,34.38 TP2.P$1
UART-RX  (via drill 0.3)
  Top 0.152: U5.RXI-0 38.5,23.3 37.2,22 v36.9,22 | J2.3 5.9,21.87 v5.9,22.5
  Bottom 0.152: v36.9,22 36.53,22.37 35.28,22.37 35.05,22.59 17.67,22.59 14.29,25.97 14.29,27.7 12.52,29.48 6.35,29.48 5.9,29.48 | v5.9,22.5 5.9,29.21 5.9,29.48 | 5.9,29.48 4.81,29.48 TP6.P$1
UART-TX  (via drill 0.3)
  Top 0.152: U5.TXO-0 v35.5,22.9 | J2.2 5.79,23.81 5.1,24.5 v5.1,25.2
  Bottom 0.152: v35.5,22.9 17.8,22.9 14.6,26.1 14.6,28 12.8,29.8 6.2,29.8 4.62,31.38 2.8,31.38 | v5.1,25.2 4.61,25.7 4.61,26.53 2.8,28.33 2.8,31.38 | TP5.P$1 2.8,32.01 2.8,31.38
V_BATT  (via drill 0.3)
  Top 0.152: v10,12.2 9.85,12.35 D1.A
  Bottom 0.152: BT1.1 12.05,10.15 v10,12.2
VDD  (via drill 0.3)
  Top 0.152: J4.2 v36.17,28.5 | U3.1 25.55,30.15 25.9,30.5 28,30.5 C22.1 28.5,32.3 29.95,33.75 J5.1 31.11,35 | R27.2 10.62,21.5 10.93,21.2 10.93,18.87 11.3,18.5 D2.C 13.7,18.5 16.53,21.33 16.53,27.87 16,28.4 R13.2 | 20.75,11.5 U2.9 U2.2 19.25,11 | 20.75,11.5 U2.10 | U2.3 19.25,11 | 15.15,11 R12.2 15.15,14.43 15.22,14.5 | 15.15,11 R14.2 10,10 8.5,8.5 C1.1 8.5,4.5 8.3,4.3 E2.2 8.3,3.5 9.3,2.5 E2.5 | 20.75,11.5 C20.1 22.85,11.85 C21.1 24.85,12.7 C4.1 | J6.11 19.25,35.4 19.53,35.68 19.53,37.47 19.5,37.5 | 31.11,35 31.11,36.48 30.1,37.5 19.5,37.5 | 15.8,37.5 10.7,37.5 E1.5 9.3,35.6 9.5,35.4 C18.1 9.5,34.1 13.45,30.15 R15.2 R13.2 | 15.8,37.5 19.5,37.5 | J6.4 15.75,37.45 15.8,37.5 | v34,31.85 34,34.2 33.2,35 31.11,35 | 15.15,11 19.25,11 | R10.2 16.85,30.15 R13.2
  Top 0.305: D2.C D1.C 13.22,16.5 15.22,14.5 v17.14,14.5 R26.1 R25.1 24.9,14.5 | 24.9,14.5 25.3,14.5 25.75,14.95 26.03,14.95 26.38,15.3 C11.1 C2.2 27.48,15.9 28.09,16.51 U5.VDD@37 28.63,16.5 29.13,17 U5.VDD@36 | C4.1 24.85,14.45 24.9,14.5
  Bottom 0.152: v36.17,28.5 36.67,29 39.3,29 | 39.3,29 39.3,30.7 38.15,31.85 R24.2 v34,31.85 | R23.2 38.95,26.15 39.3,26.5 39.3,29
  Bottom 0.305: J3.1 19.05,1.27 16.51,3.81 16.51,8.17 16.69,8.35 16.69,14.04 v17.14,14.5
X0
  Top 0.152: U5.XO 26.4,18 26.1,18.3 25.05,18.3 Y2.P$1 23.95,18.25 23.7,18.5 C10.2
~44
  Top 0.152: J3.5 33.27,1.27 35,3 35,8 39,12 39,14.09 38.84,14.26 38.84,14.7 39,14.86 U5.~D44
~45
  Top 0.152: U5.~D45 33,7 31.8,5.8 31.8,2.59 J3.4
~A31
  Top 0.152: U5.~AD31 32,7.5 29.3,4.8 29.3,2.63 J3.3
~AD33/SWO  (via drill 0.3)
  Top 0.152: U5.~AD33/SWO v30.4,20
  Bottom 0.152: v30.4,20 30.5,20 31.66,21.16 37.25,21.16 37.74,21.65 37.74,22.85 36.54,24.04 34.9,24.04 33.4,25.54 33.4,30.2 J5.6

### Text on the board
Bottom: v20
tDocu: Jim Lindblom

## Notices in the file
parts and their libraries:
SparkFun-Aesthetics: Licensing: Creative Commons ShareAlike 4.0 International - https://creativecommons.org/licenses/by-sa/4.0
SparkFun-Aesthetics: Released under the Creative Commons Attribution Share-Alike 4.0 License
SparkFun-Aesthetics: https://creativecommons.org/licenses/by-sa/4.0
